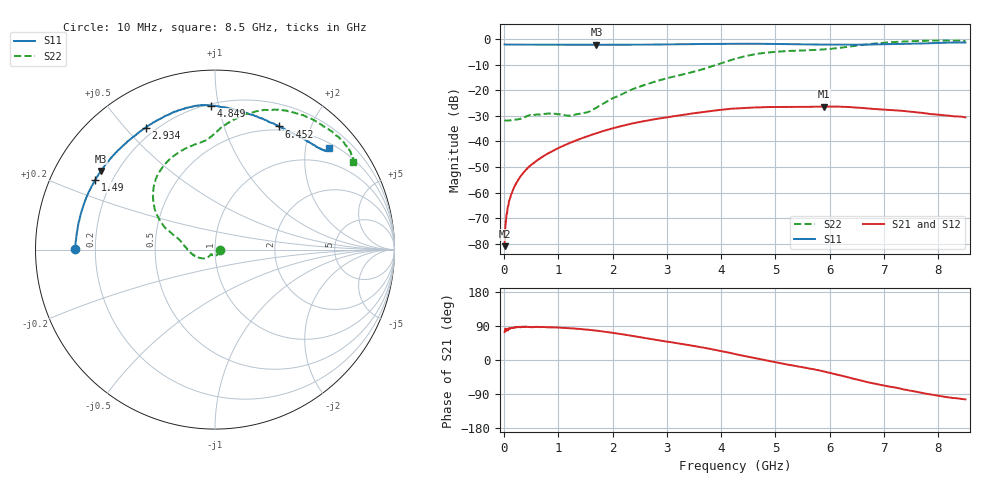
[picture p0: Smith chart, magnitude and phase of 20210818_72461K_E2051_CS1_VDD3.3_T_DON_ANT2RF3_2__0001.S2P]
!Agilent Technologies,E5071C,MY46417908,A.11.23
!Date: Wed Aug 18 14:30:16 2021
!Data & Calibration Information:
!Freq	S11:SOLT2(ON)	S21:SOLT2(ON)	S12:SOLT2(ON)	S22:SOLT2(ON)
!PortZ  Port1:50+j0  Port2:50+j0
!Above PortZ is port z conversion or system Z0 setting when saving the data.
!When reading, reference impedance value at option line is always used.
# Hz S dB R 50
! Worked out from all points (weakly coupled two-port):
!   1601 points, 10 MHz to 8.5 GHz, reference 50 ohm
!   highest |S21| = -26.37 dB at 5.895 GHz (marker M1); lowest = -80.9 dB at 10 MHz (marker M2)
!   lowest |S11| = -2.3 dB at 1.703 GHz (marker M3), VSWR 7.71, Z = 7.1 + j15.3 ohm
!   |S11| at or under -10 dB: nowhere
!   |S22| runs from -31.9 to -0.6 dB; largest |S21 - S12| = 0.00022
!   S11 on the Smith chart (normalised r, x): 10 MHz: 0.12, +0.00; 1.49 GHz: 0.14, +0.27; 2.934 GHz: 0.16, +0.57; 4.849 GHz: 0.21, +0.95; 6.452 GHz: 0.45, +1.55; 8.5 GHz: 0.60, +2.50
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1e7  -2.14 179.7  -80.88 73.8  -81.01 72.9  -31.61 -2.8
6.836875e7  -2.18 178.5  -65.69 81.0  -65.78 81.1  -31.85 -11.2
1.16125e8  -2.18 177.5  -61.83 83.4  -61.66 83.1  -31.77 -17.7
2.063312e8  -2.20 175.7  -56.92 86.2  -57.04 86.5  -31.48 -30.5
3.389875e8  -2.21 173.0  -52.73 86.9  -52.67 87.8  -30.90 -53.4
7.581812e8  -2.24 164.4  -45.29 87.0  -45.33 86.7  -29.20 -99.5
1.203906e9  -2.23 155.5  -40.65 83.9  -40.67 83.9  -29.94 -127.9
1.426769e9  -2.25 151.0  -38.81 81.4  -38.82 81.4  -29.05 -131.0
1.490444e9  -2.25 149.7  -38.32 80.6  -38.33 80.4  -28.82 -130.7
1.702694e9  -2.27 145.4  -36.77 77.6  -36.77 77.4  -26.79 -131.0
2.34475e9  -2.24 131.8  -33.08 64.0  -33.08 63.9  -19.84 -153.9
2.843538e9  -2.15 121.4  -31.09 52.1  -31.09 52.1  -16.23 179.2
2.933744e9  -2.14 119.6  -30.82 50.1  -30.81 50.1  -15.75 175.4
3.809275e9  -1.92 105.0  -28.10 29.1  -28.11 29.1  -10.80 157.3
4.255e9  -1.87 98.8  -27.13 15.8  -27.13 15.7  -7.77 145.6
4.8493e9  -1.91 91.7  -26.58 -1.4  -26.59 -1.5  -5.31 122.9
5.671769e9  -2.11 78.7  -26.47 -23.6  -26.46 -23.6  -4.35 96.2
5.894631e9  -2.16 74.2  -26.37 -30.3  -26.40 -30.3  -4.05 92.4
6.451788e9  -2.24 62.6  -26.72 -50.0  -26.73 -50.1  -2.72 81.8
7.088538e9  -2.02 50.5  -27.73 -69.9  -27.75 -70.0  -1.31 64.8
7.937538e9  -1.56 41.4  -29.43 -92.6  -29.41 -92.7  -0.62 41.9
8.5e9  -1.39 41.7  -30.59 -104.0  -30.56 -104.2  -0.80 32.5
